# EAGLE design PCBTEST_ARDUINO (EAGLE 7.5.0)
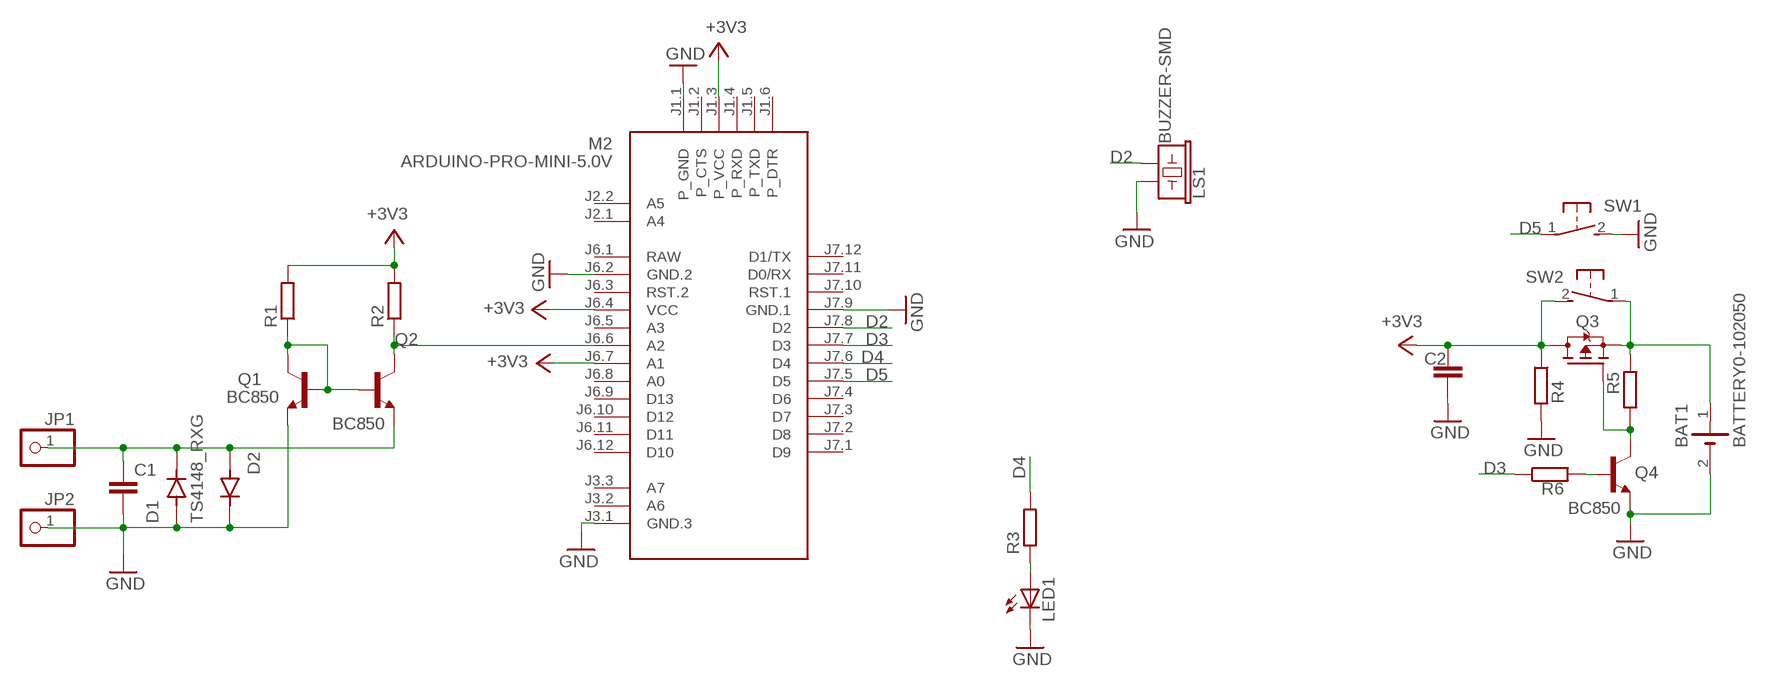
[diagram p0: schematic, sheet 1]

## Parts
BAT1  BATTERY0-102050  [BATTERY102050]
C1  C-EUC1206  [C1206]
C2  C-EUC1206  [C1206]
D1  TS4148_RXG  [DIO_TS4148_RXG]
D2  TS4148_RXG  [DIO_TS4148_RXG]
JP1  PINHD-1X1CB  [1X01-CLEANBIG]
JP2  PINHD-1X1CB  [1X01-CLEANBIG]
LED1  LED5MM  [LED5MM]
LS1  BUZZER-SMD  [BUZZER-CCV]
M2  ARDUINO-PRO-MINI-5.0V  [ARDUINO-PRO-MINI]
Q1  BC850  [SOT23]
Q2  BC850  [SOT23]
Q3  STR2P3LLH6  [SOT23]
Q4  BC850  [SOT23]
R1  R-EU_R1206  [R1206]
R2  R-EU_R1206  [R1206]
R3  R-EU_R1206  [R1206]
R4  R-EU_R1206  [R1206]
R5  R-EU_R1206  [R1206]
R6  R-EU_R1206  [R1206]
SW1  31-XX  [B3F-31XX]
SW2  31-XX  [B3F-31XX]

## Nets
+3V3: C2.2 M2.J1.3(P_VCC) M2.J6.4(VCC) M2.J6.7(A1) Q3.1(D) R1.2 R2.2 R4.1 SW2.2(S)
D2: LS1.- M2.J7.8(D2)
D3: M2.J7.7(D3) R6.1
D4: M2.J7.6(D4) R3.2
D5: M2.J7.5(D5) SW1.1(P)
GND: BAT1.2(-) C1.2 C2.1 D1.A D2.C(K) JP2.1 LED1.K(C) LS1.+ M2.J1.1(P_GND) M2.J3.1(GND.3) M2.J6.2(GND.2) M2.J7.9(GND.1) Q1.2(E) Q4.2(E) R4.2 SW1.2(S)
N$2: Q4.1(B) R6.2
N$3: LED1.A R3.1
N$4: C1.1 D1.C(K) D2.A JP1.1 Q2.2(E)
N$5: M2.J6.6(A2) Q2.3(C) R2.1
N$6: Q1.1(B) Q1.3(C) Q2.1(B) R1.1
N$15: BAT1.1(+) Q3.3(S) R5.2 SW2.1(P)
N$17: Q3.2(G) Q4.3(C) R5.1
Unconnected: M2.J1.2(P_CTS) M2.J1.4(P_RXD) M2.J1.5(P_TXD) M2.J1.6(P_DTR) M2.J2.1(A4) M2.J2.2(A5) M2.J3.2(A6) M2.J3.3(A7) M2.J6.3(RST.2) M2.J6.5(A3) M2.J6.8(A0) M2.J6.9(D13) M2.J6.10(D12) M2.J6.11(D11) M2.J6.12(D10) M2.J7.1(D9) M2.J7.2(D8) M2.J7.3(D7) M2.J7.4(D6) M2.J7.10(RST.1) M2.J7.11(D0/RX) M2.J7.12(D1/TX)

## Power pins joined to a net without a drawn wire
RAW: M2.J6.1(RAW)

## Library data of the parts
BAT1 = battery:BATTERY0-102050
C1 C2 = rcl:C-EU: CAPACITOR, European symbol
D1 D2 = TS4148_RXG:TS4148_RXG: Check availability Check availability Check availability; AVAILABILITY: In Stock; CHECK_PRICES: https://www.snapeda.com/parts/TS4148%20RXG/Taiwan+Semiconductor/view-part/?ref=eda; DESCRIPTION: 1206 (Ceramics) 75V 0.15A Switching Diode & Array; MF: Taiwan Semiconductor; MP: TS4148 RXG; PACKAGE: 1206-2 Taiwan Semiconductor; PRICE: None; SNAPEDA_LINK: https://www.snapeda.com/parts/TS4148%20RXG/Taiwan+Semiconductor/view-part/?ref=snap
JP1 JP2 = adafruit:PINHD-1X1: Pin header 1x1 for 0.1" spacing
LED1 = led:LED: LED
LS1 = SparkFun-Electromechanical:BUZZER: Buzzer; PROD_ID: COMP-08568
M2 = diy-modules:ARDUINO-PRO-MINI-*: Arduino Pro Mini and compatible devices More details available here: https://www.arduino.cc/en/Main/ArduinoBoardProMini Click here to find device on ebay.com
Q1 Q2 Q4 = transistor:BC850: NPN TRANSISTOR
Q3 = transistor-fet:STR2P3LLH6
R1-R6 = rcl:R-EU_: RESISTOR, European symbol
SW1 SW2 = switch-omron:31-XX: OMRON SWITCH; MPN: B3F-3100; OC_FARNELL: 959704; OC_NEWARK: 36M3582

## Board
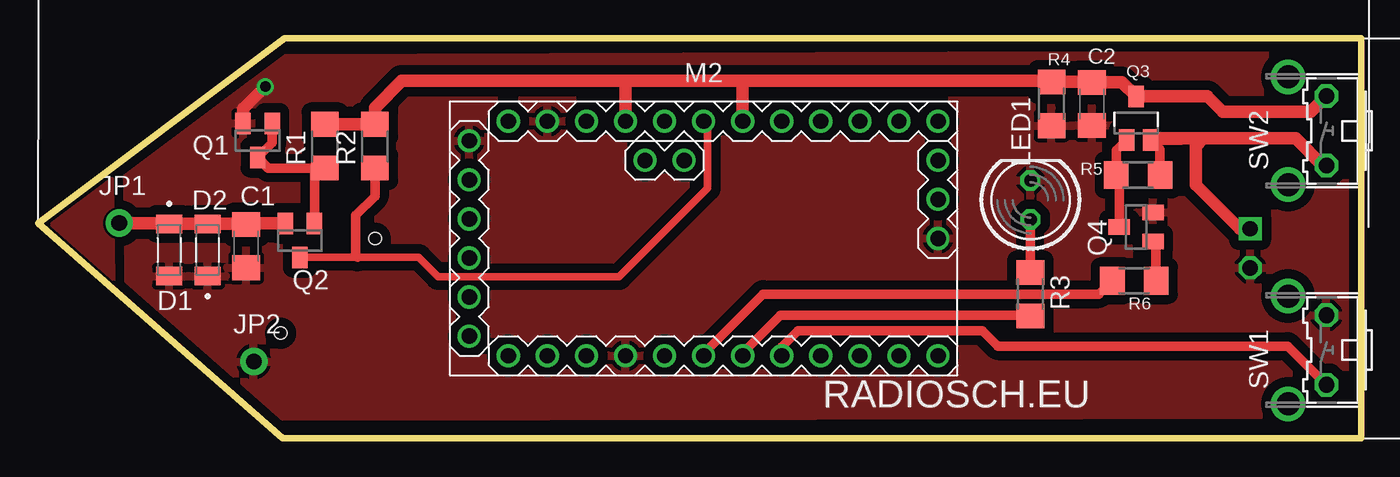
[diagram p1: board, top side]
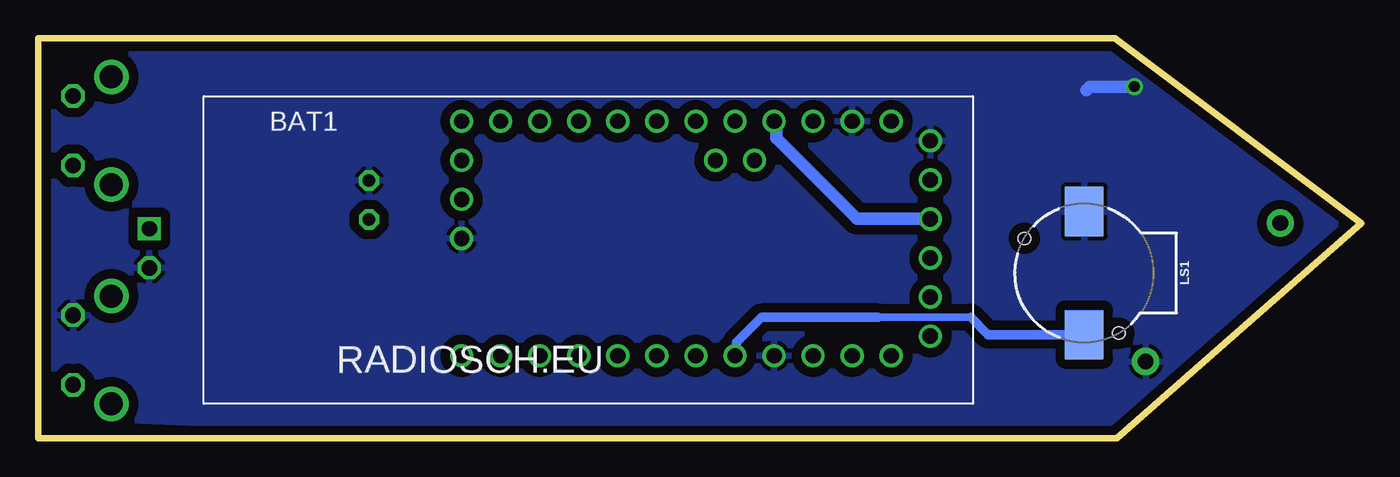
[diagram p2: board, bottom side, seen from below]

Size 86 x 26 mm. Coordinates in mm from the lower left corner, seen from the top.
Outline: 0,14 16,26 86,26 86,0 15.88,0 0,14
Copper layers (1*16): Top 0.035mm / dielectric 1.5mm / Bottom 0.035mm
Design rules "default *": minimum track width 10mil, minimum drill 20mil, track to track 6mil, track to pad 6mil, pad to pad 6mil, via to via 6mil, smd to smd 6mil, copper to edge 6mil, drill to drill 6mil, minimum pad ring 10mil, minimum via ring 8mil, stop-mask expansion 4mil, vias tented up to drill 20mil, thermal gap 10mil

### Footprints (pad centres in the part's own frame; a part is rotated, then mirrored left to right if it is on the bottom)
BATTERY102050 = drill 1 square: 1 -2.54,-7.62 | drill 1 octagon: 2 -2.54,-10.16
C1206 = smd 1.6 x 1.8: 1 -1.4,0; 2 1.4,0
DIO_TS4148_RXG = smd 1.2 x 1.7: A 1.7,0; C -1.7,0
1X01-CLEANBIG = drill 1.016 pad 1.778: 1 0,0
LED5MM = drill 0.813 octagon: A -1.27,0; K 1.27,0
BUZZER-CCV = smd 3.2 x 2.5: + 4,0; - -4,0 | hole 0.8: -3.9,-2.25; 2.25,3.9
ARDUINO-PRO-MINI = drill 1: J1.1 -15.24,6.35; J1.2 -15.24,3.81; J1.3 -15.24,1.27; J1.4 -15.24,-1.27; J1.5 -15.24,-3.81; J1.6 -15.24,-6.35; J2.1 -1.27,5.08; J2.2 -3.81,5.08; J3.1 15.24,0; J3.2 15.24,2.54; J3.3 15.24,5.08; J6.1 -12.7,7.62; J6.2 -10.16,7.62; J6.3 -7.62,7.62; J6.4 -5.08,7.62; J6.5 -2.54,7.62; J6.6 0,7.62; J6.7 2.54,7.62; J6.8 5.08,7.62; J6.9 7.62,7.62; J6.10 10.16,7.62; J6.11 12.7,7.62; J6.12 15.24,7.62; J7.1 15.24,-7.62; J7.2 12.7,-7.62; J7.3 10.16,-7.62; J7.4 7.62,-7.62; J7.5 5.08,-7.62; J7.6 2.54,-7.62; J7.7 0,-7.62; J7.8 -2.54,-7.62; J7.9 -5.08,-7.62; J7.10 -7.62,-7.62; J7.11 -10.16,-7.62; J7.12 -12.7,-7.62
SOT23 = smd 1 x 1.4: 1 -0.95,-1.1; 2 0.95,-1.1; 3 0,1.1
SOT23' = smd 1 x 1.4: 1 0,1.735; 2 -0.632,-1.1; 3 0.95,-1.1
R1206 = smd 1.6 x 1.803: 1 -1.422,0; 2 1.422,0
B3F-31XX = drill 1.016 octagon: 1 -2.261,-1.245; 2 2.261,-1.245 | drill 1.499 pad 2.159: 3 -3.505,1.245; 4 3.505,1.245

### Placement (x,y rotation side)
BAT1  76.25,21.25 0 bottom
C1  13.5,12.5 270 top
C2  68.5,21.75 90 top
D1  8.5,12.25 270 top
D2  11,12.25 90 top
JP1  5.25,14 0 top
JP2  14,5 0 top
LED1  64.5,15.5 90 top
LS1  18,10.75 90 bottom
M2  43.25,13 0 top
Q1  14.25,19.38 180 top
Q2  17,12.88 180 top
Q3  STR2P3LLH6  [SOT23']  71.38,20.5 0 top
Q4  71.38,13.75 90 top
R1  18.62,19 90 top
R2  21.88,19 90 top
R3  64.5,9.38 270 top
R4  65.88,21.75 270 top
R5  71.5,17.12 0 top
R6  71.25,10.25 0 top
SW1  82.5,5.75 90 top
SW2  82.5,20 90 top

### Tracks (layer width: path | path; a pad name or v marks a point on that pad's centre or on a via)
+3V3
  Top 0.813: R2.2 21.88,21.12 | 38,23.25 23.62,23.25 21.88,21.5 21.88,21.12 | 38,23.25 45.5,23.25 | 45.5,23.25 65.8,23.25 R4.1 | R4.1 65.7,23.17 | R4.1 68.48,23.17 C2.2 70.46,23.15 Q3.1 76.02,22.23 77,21.25 82.73,21.25 SW2.2 | M2.J6.4 38.17,23.08 38,23.25 | M2.J6.7 45.79,22.96 45.5,23.25 | R1.2 21.17,20.42 21.88,21.12
  Bottom 0.813: M2.J1.3 32.77,14.27 38,19.5 38,20.45 M2.J6.4
D2
  Bottom 0.5: 25.38,7.88 31.38,7.88
  Bottom 0.61: LS1.- 24.25,6.75 25.38,7.88 | 31.38,7.88 39,7.88 40.62,6.25 40.62,5.46 M2.J7.8
D3
  Top 0.61: M2.J7.7 43.25,5.5 47.12,9.38 68.95,9.38 R6.1
D4
  Top 0.61: M2.J7.6 45.79,5.54 48.25,8 64.45,8 R3.2
D5
  Top 0.61: M2.J7.5 48.33,5.96 49.38,7 61.38,7 62.38,6 81.23,6 SW1.1
GND  (via drill 0.7)
  Top 0.813: Q1.2 13.3,21.43 v14.75,22.88
  Bottom 0.813: v14.75,22.88 17.62,22.88 17.88,22.62
  pour Top (isolate 0.61, rank 2): 0.5,14.25 16,24.75 85,25 85.25,1.5 15.88,1.38
  pour Bottom (isolate 0.61): -0.12,13.88 16.12,25 85.12,25 85.38,1.38 71.88,0.88 16.38,1 0,13.88
N$1
  pour Top: 0.75,13.88 4.62,16.75 4.75,16.88 4.88,10.25
N$2
  Top 0.61: R6.2 72.67,12.6 Q4.1
N$3
  Top 0.61: R3.1 LED1.A
N$4
  Top 0.813: JP1.1 8.45,14 D1.C D2.A 13.45,13.95 C1.1 13.57,13.97 Q2.2
N$5
  Top 0.5: Q2.3 20.75,11.78 24.73,11.78 26,10.5 37.75,10.5 43.5,16.25 43.5,20.37 M2.J6.6
  Top 0.61: R2.1 21.88,15.75 20.62,14.5 20.62,11.9 20.75,11.78
N$6
  Top 0.61: R1.1 18.12,17.58 | 18.12,17.58 14.95,17.58 Q1.3 15.2,19.23 Q1.1 | Q2.1 17.95,17.4 18.12,17.58
N$15
  Top 0.61: 74.32,19.4 Q3.3 72.92,18.8 R5.2
  Top 0.813: BAT1.1 78.12,13.63 75.25,16.5 75.25,19 | 75.25,19 75.25,19.5 | 76,19.5 75.25,19.5 | 75.25,19.5 72.42,19.5 Q3.3 | SW2.1 83.51,17.74 81.75,19.5 75.75,19.5 75.25,19
N$17
  Top 0.61: Q4.3 70.28,16.93 R5.1 70.08,18.74 Q3.2

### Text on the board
tPlace: RADIOSCH.EU
bPlace: RADIOSCH.EU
